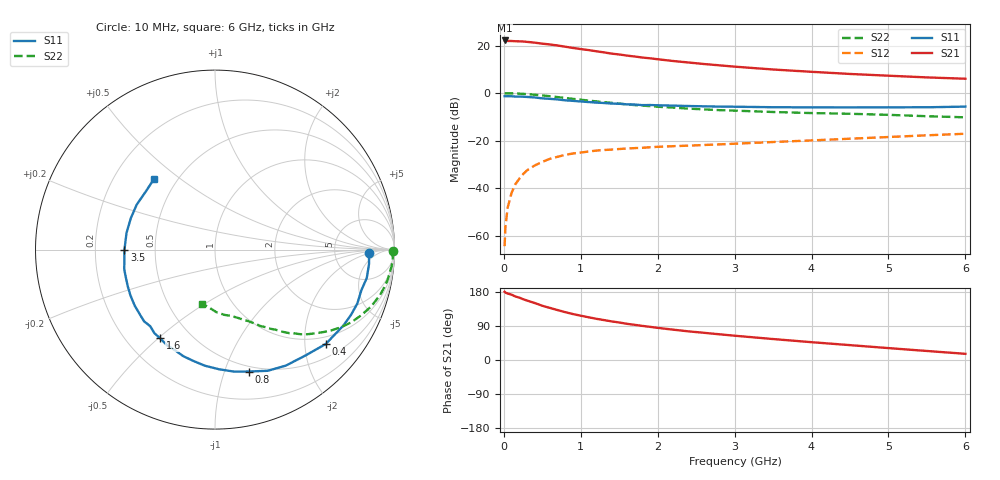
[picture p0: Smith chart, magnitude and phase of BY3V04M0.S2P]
! SIEMENS Small Signal Semiconductors
! BFY420
! Si NPN RF SIEGET Grounded Emitter Transistor in MICRO-X
! VCE = 3 V  IC = 4 mA
! Common Emitter S-Parameters:  October  1996
# GHz  S  MA  R  50
!  f  S11  S21  S12  S22
! GHz  MAG  ANG  MAG  ANG  MAG  ANG  MAG  ANG
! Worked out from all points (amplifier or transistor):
!   36 points, 10 MHz to 6 GHz, reference 50 ohm
!   highest |S21| = 22.2 dB at 10 MHz (marker M1)
!   |S21| within 3 dB of that: start of sweep to 868.3 MHz
!   unconditionally stable (mu >= 1): 3.377 GHz to end of sweep
!   at 250 MHz: K = 0.11, MSG = 27.9 dB, |S12| = -34.1 dB
!   at 1.4 GHz: K = 0.46, MSG = 20.2 dB, |S12| = -23.8 dB
!   at 6 GHz: K = 1.16, MAG = 9.2 dB, |S12| = -17.1 dB
!   S11 on the Smith chart (normalised r, x): 10 MHz: 13, -2; 400 MHz: 0.81, -2.48; 800 MHz: 0.45, -1.22; 1.6 GHz: 0.34, -0.51; 3.5 GHz: 0.33, -0.00; 6 GHz: 0.37, +0.40
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0.01  0.8605 -1.1  12.85 180.0  0.0006 86.1  0.9921 -0.5
0.02  0.8583 -2.2  12.79 177.9  0.0015 80.6  0.9871 -1.0
0.05  0.862 -5.2  12.54 175.4  0.0039 88.5  0.9918 -2.6
0.1  0.8603 -10.6  12.51 172.4  0.0079 84.6  0.9886 -5.2
0.15  0.8463 -15.5  12.39 167.6  0.0121 79.1  0.9815 -7.8
0.2  0.848 -20.8  12.3 164.7  0.0157 79.6  0.9755 -10.2
0.25  0.8404 -25.7  12.23 160.5  0.0197 74.7  0.965 -12.8
0.4  0.8106 -40.5  11.56 150.5  0.0299 68.4  0.9265 -19.9
0.5  0.7756 -49.6  11 143.1  0.0358 64.2  0.8941 -24.1
0.6  0.7573 -58.6  10.58 137.4  0.0414 59.7  0.8604 -28.1
0.7  0.7363 -66.5  10.07 131.6  0.0458 56.4  0.8251 -31.6
0.8  0.7052 -74.4  9.473 126.2  0.0503 52.9  0.789 -34.8
0.9  0.6878 -81.2  8.926 121.2  0.0536 50.0  0.7573 -37.4
1.1  0.6494 -95.0  8.067 112.8  0.059 46.1  0.6979 -42.5
1.4  0.6033 -111.7  6.793 101.9  0.0647 40.8  0.6237 -48.3
1.6  0.581 -121.8  6.174 95.5  0.0682 38.3  0.5791 -51.6
2.2  0.5456 -145.1  4.747 80.1  0.0764 34.4  0.4957 -59.2
2.8  0.5204 -162.7  3.85 67.9  0.0834 32.2  0.4382 -65.2
3.5  0.5049 -179.6  3.143 55.3  0.0935 30.9  0.4006 -71.6
4.5  0.5006 159.6  2.533 39.2  0.1097 28.1  0.3676 -81.7
5.5  0.5037 139.7  2.143 23.8  0.1295 24.0  0.3265 -95.1
6  0.5201 130.8  2.009 16.3  0.1396 21.3  0.3095 -103.2
